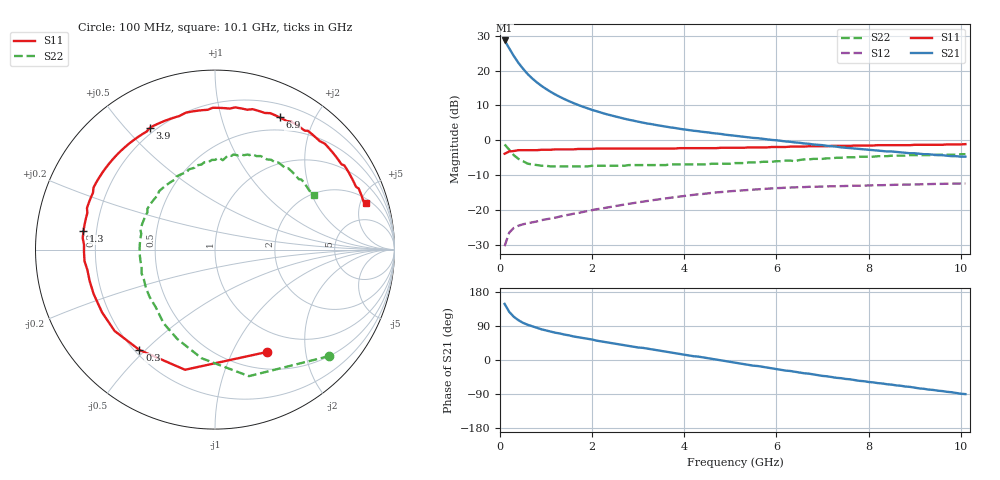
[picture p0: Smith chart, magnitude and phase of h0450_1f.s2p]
!HBFP-0450
!S and NOISE PARAMETERS at Vce=1V  Ic=20mA.  LAST UPDATED  09-04-98
# GHZ S MA R  50
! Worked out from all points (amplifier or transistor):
!   101 points, 100 MHz to 10.1 GHz, reference 50 ohm
!   highest |S21| = 28.7 dB at 100 MHz (marker M1)
!   |S21| within 3 dB of that: start of sweep to 233.3 MHz
!   unconditionally stable (mu >= 1): 2.369 GHz to end of sweep
!   at 1.7 GHz: K = 0.89, MSG = 15.5 dB, |S12| = -20.9 dB
!   at 5.1 GHz: K = 1.11, MAG = 5.9 dB, |S12| = -14.6 dB
!   at 10.1 GHz: K = 1.05, MAG = 2.5 dB, |S12| = -12.4 dB
!   lowest NFmin = 1.33 dB at 1.8 GHz
!   S11 on the Smith chart (normalised r, x): 100 MHz: 0.71, -1.38; 300 MHz: 0.22, -0.48; 1.3 GHz: 0.15, +0.07; 3.9 GHz: 0.18, +0.59; 6.9 GHz: 0.34, +1.55; 10.1 GHz: 2.47, +5.64
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0.1  0.64 -63.0  27.21 148.0  0.03 63.0  0.87 -43.0
0.2  0.69 -104.0  20.98 127.0  0.047 46.0  0.73 -75.0
0.3  0.7 -127.0  16.24 114.0  0.055 37.0  0.61 -97.0
0.4  0.72 -141.0  12.95 105.0  0.059 32.0  0.54 -113.0
0.5  0.72 -151.0  10.67 98.0  0.062 30.0  0.5 -125.0
0.6  0.72 -160.0  8.95 93.0  0.064 29.0  0.46 -136.0
0.7  0.72 -166.0  7.73 89.0  0.066 28.0  0.45 -144.0
0.8  0.72 -171.0  6.8 85.0  0.068 28.0  0.44 -151.0
0.9  0.73 -175.0  6.05 81.0  0.071 28.0  0.43 -157.0
1.1  0.73 178.0  4.96 75.0  0.075 28.0  0.42 -167.0
1.3  0.74 172.0  4.2 70.0  0.08 28.0  0.42 -175.0
1.6  0.74 164.0  3.41 62.0  0.088 28.0  0.42 176.0
1.8  0.75 159.0  3.03 58.0  0.093 27.0  0.42 170.0
2.1  0.76 153.0  2.61 51.0  0.102 26.0  0.43 163.0
2.5  0.76 145.0  2.2 43.0  0.113 24.0  0.43 155.0
3.5  0.76 125.0  1.61 24.0  0.143 16.0  0.44 138.0
3.9  0.77 118.0  1.46 16.0  0.155 12.0  0.45 131.0
5.1  0.78 97.0  1.16 -7.0  0.187 -3.0  0.47 108.0
6.8  0.82 66.0  0.87 -38.0  0.214 -27.0  0.54 79.0
6.9  0.82 64.0  0.86 -40.0  0.215 -29.0  0.54 77.0
8.5  0.85 40.0  0.69 -65.0  0.228 -49.0  0.6 54.0
10.1  0.88 17.0  0.58 -90.0  0.239 -72.0  0.63 29.0
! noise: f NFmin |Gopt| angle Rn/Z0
1.8  1.33  0.5  -166  0.06
2  1.38  0.52  -163  0.06
2.5  1.5  0.55  -151  0.09
3.5  1.71  0.62  -132  0.19
4  1.85  0.65  -121  0.3
5  2.08  0.7  -102  0.59
5.5  2.21  0.72  -91  0.84
7  2.55  0.77  -63  1.81
8  2.79  0.81  -47  2.67
10  3.26  0.83  -17  4.36
